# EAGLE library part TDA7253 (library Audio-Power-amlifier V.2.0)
8W AMPLIFIER WITH MUTING
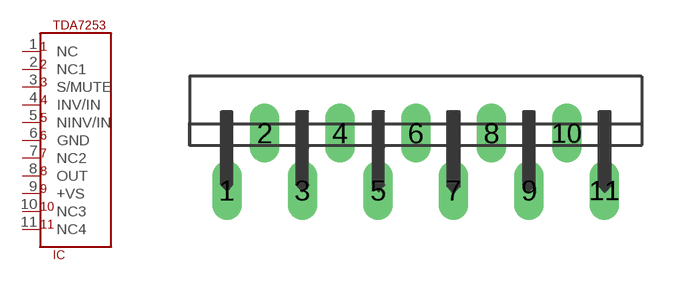
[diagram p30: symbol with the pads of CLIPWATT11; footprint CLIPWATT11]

Designator prefix IC

## TDA7253  [CLIPWATT11]
1  NC  nc
2  NC1  nc
3  S/MUTE
4  INV/IN  in
5  NINV/IN  in
6  GND  pwr
7  NC2  nc
8  OUT  out
9  +VS  pwr
10  NC3  nc
11  NC4  nc

## Footprint CLIPWATT11 (pad centres in mm)
drill 0.8 long: 1 -8.382,0; 2 -6.706,2.54; 3 -5.029,0; 4 -3.353,2.54; 5 -1.676,0; 6 0,2.54; 7 1.676,0; 8 3.353,2.54; 9 5.029,0; 10 6.706,2.54; 11 8.382,0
